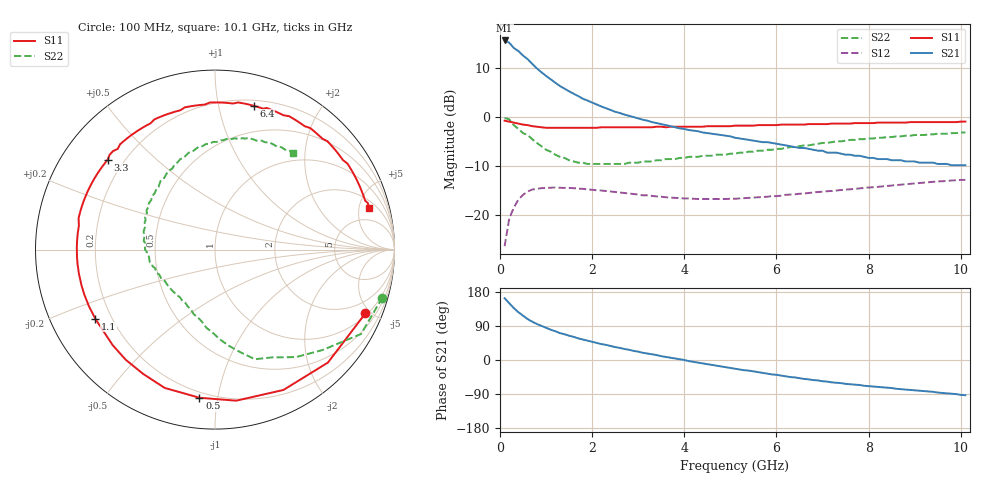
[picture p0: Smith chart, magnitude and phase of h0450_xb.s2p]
!HBFP-0450
!S and NOISE PARAMETERS at Vce=0.5V  Ic=2mA.  LAST UPDATED  09-04-98
# GHZ S MA R  50
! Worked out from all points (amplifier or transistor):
!   101 points, 100 MHz to 10.1 GHz, reference 50 ohm
!   highest |S21| = 15.5 dB at 100 MHz (marker M1)
!   |S21| within 3 dB of that: start of sweep to 491.7 MHz
!   unconditionally stable (mu >= 1): 3.2 GHz to end of sweep
!   at 1.7 GHz: K = 0.50, MSG = 9.4 dB, |S12| = -14.7 dB
!   at 5.1 GHz: K = 1.42, MAG = 2.4 dB, |S12| = -16.7 dB
!   at 10.1 GHz: K = 1.19, MAG = -1.1 dB, |S12| = -12.9 dB
!   lowest NFmin = 1.48 dB at 1.8 GHz
!   S11 on the Smith chart (normalised r, x): 100 MHz: 1.13, -4.65; 500 MHz: 0.17, -0.89; 1.1 GHz: 0.14, -0.26; 3.3 GHz: 0.14, +0.36; 6.4 GHz: 0.25, +1.27; 10.1 GHz: 2.86, +6.33
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0.1  0.91 -23.0  5.97 163.0  0.048 76.0  0.97 -16.0
0.2  0.89 -45.0  5.67 150.0  0.091 62.0  0.94 -30.0
0.3  0.87 -64.0  5 137.0  0.119 51.0  0.82 -43.0
0.4  0.85 -82.0  4.65 126.0  0.143 42.0  0.75 -53.0
0.5  0.83 -96.0  4.19 117.0  0.16 34.0  0.68 -62.0
0.6  0.82 -110.0  3.85 108.0  0.173 28.0  0.65 -70.0
0.7  0.8 -120.0  3.45 101.0  0.181 22.0  0.59 -76.0
0.8  0.79 -129.0  3.1 95.0  0.184 18.0  0.54 -82.0
0.9  0.78 -137.0  2.83 90.0  0.187 14.0  0.5 -87.0
1.1  0.77 -150.0  2.4 80.0  0.189 7.0  0.44 -96.0
1.3  0.77 -161.0  2.05 71.0  0.189 2.0  0.39 -104.0
1.8  0.77 179.0  1.52 54.0  0.184 -8.0  0.34 -122.0
2.5  0.78 159.0  1.12 34.0  0.171 -17.0  0.33 -143.0
3.3  0.78 140.0  0.88 15.0  0.156 -23.0  0.35 -163.0
3.5  0.79 136.0  0.84 10.0  0.153 -24.0  0.36 -167.0
4.2  0.79 121.0  0.72 -5.0  0.146 -26.0  0.39 178.0
5.1  0.81 102.0  0.61 -23.0  0.146 -27.0  0.42 157.0
6.4  0.83 75.0  0.49 -46.0  0.162 -32.0  0.49 125.0
6.8  0.84 68.0  0.46 -53.0  0.169 -35.0  0.52 116.0
7.6  0.85 54.0  0.41 -64.0  0.182 -41.0  0.58 99.0
8.5  0.87 40.0  0.36 -74.0  0.199 -49.0  0.62 82.0
10.1  0.89 15.0  0.32 -93.0  0.227 -70.0  0.69 51.0
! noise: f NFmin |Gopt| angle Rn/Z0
1.8  1.48  0.68  160  0.05
2  1.51  0.68  169  0.04
2.5  1.73  0.74  -174  0.03
3.5  2.18  0.77  -145  0.22
4  2.46  0.79  -133  0.43
5  2.8  0.82  -109  1.17
5.5  3.22  0.83  -97  1.81
7  3.85  0.86  -66  4.22
8  4.07  0.87  -49  5.88
10  4.83  0.84  -18  8.4
